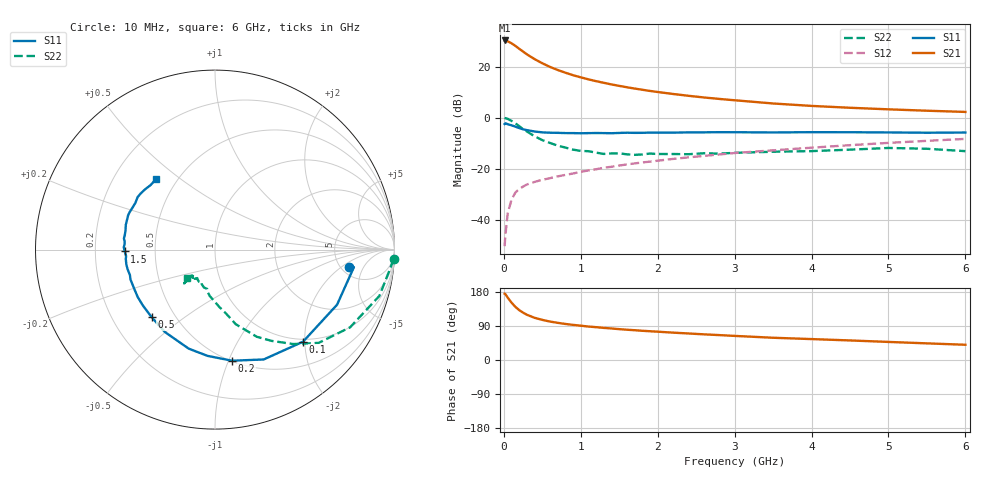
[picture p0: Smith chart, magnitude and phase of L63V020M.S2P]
!  INFINEON TECHNOLOGIES Small Signal Semiconductors
! BFR380L3 , Si-NPN RF-Transistor in TSLP-3-1
!  Vce=3 V,  Ic=20 mA
! Common Emitter S-Parameters:  07. March 2005
#  GHz  S  MA  R  50
! f  S11  S21  S12  S22
! GHz  Mag  Ang  Mag  Ang  Mag  Ang  Mag  Ang
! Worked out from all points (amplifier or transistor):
!   36 points, 10 MHz to 6 GHz, reference 50 ohm
!   highest |S21| = 30.4 dB at 10 MHz (marker M1)
!   |S21| within 3 dB of that: start of sweep to 188.2 MHz
!   unconditionally stable (mu >= 1): 1.912 GHz to 4.804 GHz
!   at 250 MHz: K = 0.37, MSG = 26.5 dB, |S12| = -27.1 dB
!   at 1.4 GHz: K = 0.95, MSG = 16.2 dB, |S12| = -19.3 dB
!   at 6 GHz: K = 0.97, MSG = 5.3 dB, |S12| = -8.3 dB
!   S11 on the Smith chart (normalised r, x): 10 MHz: 5.87, -2.62; 100 MHz: 0.95, -1.96; 200 MHz: 0.51, -1.03; 500 MHz: 0.37, -0.38; 1.5 GHz: 0.33, -0.01; 6 GHz: 0.38, +0.41
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0.01  0.7521 -7.4  32.98 175.0  0.003 77.9  0.996 -3.1
0.02  0.7801 -7.2  32.84 173.8  0.0049 84.4  0.9802 -6.5
0.05  0.7462 -24.3  31.79 164.7  0.0131 80.3  0.9518 -15.7
0.1  0.7099 -46.3  29.02 151.4  0.0247 70.5  0.8684 -29.9
0.15  0.6695 -66.1  25.82 140.2  0.0339 62.2  0.7768 -42.0
0.2  0.6263 -81.3  22.64 131.6  0.0398 58.8  0.6841 -50.3
0.25  0.5937 -94.0  19.97 125.0  0.0444 54.5  0.5975 -58.3
0.3  0.5708 -104.9  17.59 119.4  0.0489 53.2  0.5384 -64.4
0.4  0.5372 -121.4  14.18 111.3  0.0549 51.2  0.432 -74.4
0.5  0.516 -133.2  11.75 105.9  0.0604 52.0  0.3635 -80.0
0.6  0.5083 -142.2  9.959 101.4  0.065 51.9  0.3193 -85.9
0.7  0.5052 -148.5  8.679 98.1  0.0705 53.5  0.2839 -91.3
0.9  0.4995 -160.5  6.845 92.7  0.0803 56.3  0.236 -100.4
1.1  0.4993 -167.4  5.68 88.3  0.0922 57.9  0.2201 -106.2
1.5  0.5029 -178.8  4.226 81.4  0.1151 60.8  0.1999 -116.4
1.8  0.5056 174.7  3.548 77.1  0.1324 61.8  0.1898 -121.8
2.2  0.51 167.8  2.931 72.2  0.1552 62.7  0.1938 -125.4
2.8  0.5204 158.5  2.342 65.7  0.1898 63.5  0.1972 -132.5
3.5  0.5141 149.6  1.906 58.7  0.2289 62.3  0.2149 -132.3
4.5  0.5192 143.1  1.57 51.6  0.2892 61.4  0.2361 -132.4
5.5  0.5078 134.9  1.374 43.9  0.3517 58.2  0.2458 -132.5
6  0.5125 129.7  1.301 40.2  0.3844 56.2  0.2207 -134.3
